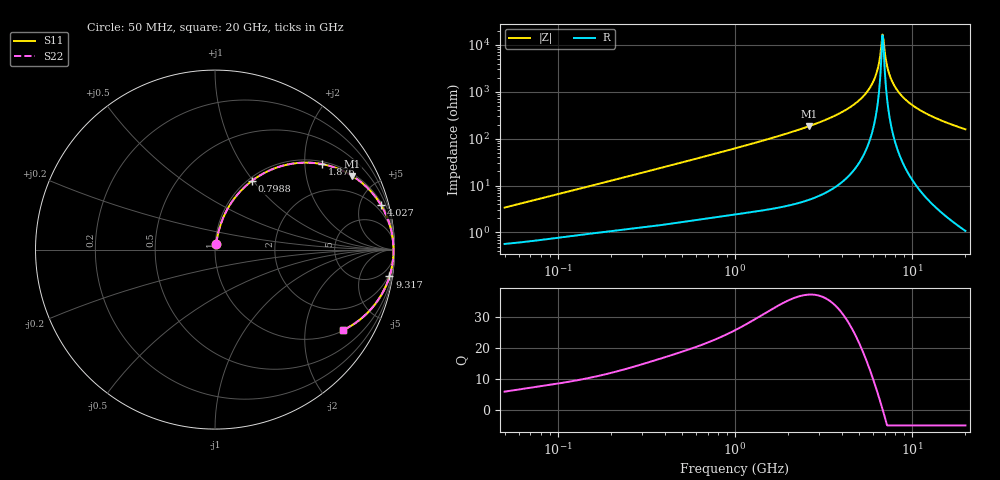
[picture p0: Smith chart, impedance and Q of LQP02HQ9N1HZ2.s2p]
!Murata Part Number: LQP02HQ9N1HZ2
!These Parameters are Measured in Series Mode Connection
!  o--[Z]--o
!Port1  Port2
!  o-------o
!Freq. Start=50[MHz] Stop=20[GHz], 401[Steps]
# Hz S RI R 50
!Freq.(Hz) S11(Real) S11(Imag) S21(Real) S21(Imag) S12(Real) S12(Imag) S22(Real) S22(Imag)
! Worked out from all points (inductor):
!   401 points, 50 MHz to 20 GHz, reference 50 ohm
!   read as one part in series: L = 10.6 nH near 51.52 MHz
!   highest Q = 37.1 at 2.608 GHz (marker M1), where L = 11.2 nH
!   self-resonance near 6.802 GHz
!   S11 on the Smith chart (normalised r, x): 50 MHz: 1.01, +0.07; 798.8 MHz: 1.04, +0.99; 1.876 GHz: 1.07, +2.44; 4.027 GHz: 1.24, +7.40; 9.317 GHz: 1, -13; 20 GHz: 1.02, -3.16
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5e7  0.00677 0.033  0.9932 -0.033  0.9932 -0.033  0.00677 0.033
1.364002e8  0.0163 0.0856  0.9837 -0.0856  0.9837 -0.0856  0.0163 0.0856
3.721004e8  0.063 0.2143  0.937 -0.2143  0.937 -0.2143  0.063 0.2143
7.987718e8  0.2066 0.3837  0.7934 -0.3837  0.7934 -0.3837  0.2066 0.3837
1e9  0.2858 0.4327  0.7142 -0.4327  0.7142 -0.4327  0.2858 0.4327
1.875929e9  0.5961 0.4764  0.4039 -0.4764  0.4039 -0.4764  0.5961 0.4764
2.608132e9  0.7649 0.4108  0.2351 -0.4108  0.2351 -0.4108  0.7649 0.4108
2.728004e9  0.7855 0.3972  0.2145 -0.3972  0.2145 -0.3972  0.7855 0.3972
4.026975e9  0.9252 0.2475  0.0748 -0.2475  0.0748 -0.2475  0.9252 0.2475
4.966507e9  0.969 0.1521  0.031 -0.1521  0.031 -0.1521  0.969 0.1521
5.769027e9  0.987 0.0811  0.013 -0.0811  0.013 -0.0811  0.987 0.0811
6.311513e9  0.9926 0.0379  0.00742 -0.0379  0.00742 -0.0379  0.9926 0.0379
6.701223e9  0.9942 0.00896  0.00584 -0.00896  0.00584 -0.00896  0.9942 0.00896
6.802353e9  0.9943 0.00172  0.00572 -0.00172  0.00572 -0.00172  0.9943 0.00172
6.905011e9  0.9943 -0.00552  0.0057 0.00552  0.0057 0.00552  0.9943 -0.00552
7.009217e9  0.9942 -0.0128  0.00579 0.0128  0.00579 0.0128  0.9942 -0.0128
7.222371e9  0.9937 -0.0272  0.00628 0.0272  0.00628 0.0272  0.9937 -0.0272
7.442007e9  0.9928 -0.0417  0.00721 0.0417  0.00721 0.0417  0.9928 -0.0417
8.141811e9  0.9874 -0.085  0.0126 0.085  0.0126 0.085  0.9874 -0.085
9.316812e9  0.9721 -0.1494  0.0279 0.1494  0.0279 0.1494  0.9721 -0.1494
1.276073e10  0.9005 -0.2924  0.0995 0.2924  0.0995 0.2924  0.9005 -0.2924
2e10  0.7127 -0.4491  0.2873 0.4491  0.2873 0.4491  0.7127 -0.4491
